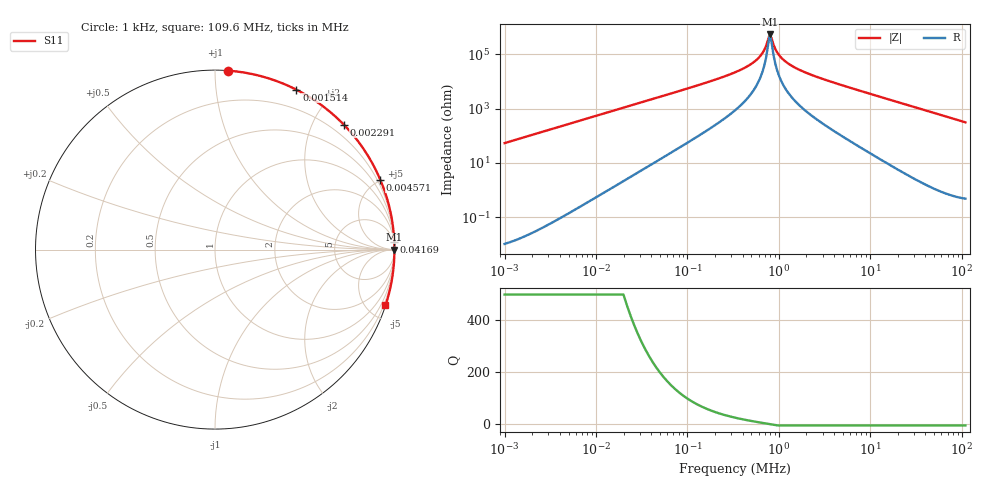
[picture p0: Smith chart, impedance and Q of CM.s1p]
! EM Consulting and Software
! Touchstone file was created on 2026-03-09  16:25:52
# HZ S RI R 50.0000
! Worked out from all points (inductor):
!   253 points, 1 kHz to 109.6 MHz, reference 50 ohm
!   read as one part to ground: L = 8.57 mH near 1.047 kHz
!   highest |Z| = 531 kohm at 794.3 kHz (marker M1)
!   self-resonance near 794.3 kHz
!   S11 on the Smith chart (normalised r, x): 1 kHz: 0.00, +1.08; 1.514 kHz: 0.00, +1.63; 2.291 kHz: 0.00, +2.47; 4.571 kHz: 0.00, +4.92; 41.69 kHz: 0, +45; 109.6 MHz: 0.01, -6.26
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1000  0.0743 0.997
1202.264  0.253 0.9673
1513.561  0.4533 0.8911
1819.701  0.587 0.8094
1995.262  0.6441 0.7647
2290.868  0.7178 0.6959
2630.268  0.7784 0.6275
3162.278  0.8412 0.5404
3630.781  0.8771 0.4798
4365.158  0.9133 0.4068
4570.882  0.9206 0.39
6309.573  0.9575 0.2879
8709.636  0.9774 0.2107
12589.25  0.989 0.1466
18197.01  0.9946 0.1017
26302.68  0.9973 0.0704
41686.94  0.9988 0.0444
79432.82  0.9995 0.0231
331131.1  0.9998 0.00465
794328.2  0.9998 3.34e-05
1445440  0.9998 -0.00291
6025596  0.9997 -0.0172
1.380384e7  0.999 -0.0399
2.630268e7  0.9969 -0.076
3.981072e7  0.9932 -0.1146
5.754399e7  0.9861 -0.1648
7.943282e7  0.9737 -0.2262
1.096478e8  0.9498 -0.3114
